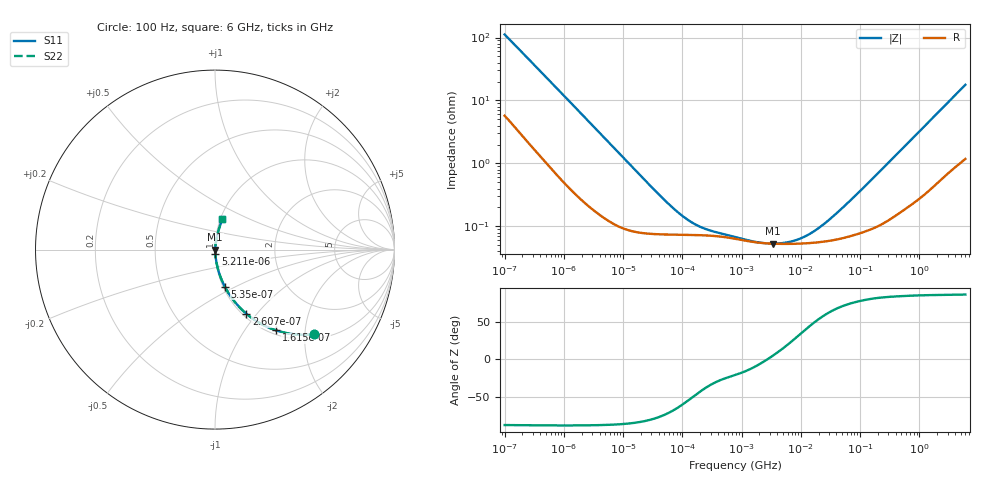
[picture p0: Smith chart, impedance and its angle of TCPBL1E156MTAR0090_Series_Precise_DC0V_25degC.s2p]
! TCPBL1E156MTAR0090 Polymer Tantalum Capacitor Sparameter Model
! Model Generated by Samsung Electro-Mechanics
! Samsung Sparameter Version 5.0
! Date : Oct-10-2024
! Products : Polymer Tantalum Capacitor
! Characteristics :
!  Nominal Capacitance = 15uF
!  Capacitance Tolerance = +/-20%
!  ESR = 90 mohm max at 100kHz
!  Rated Voltage = 25Vdc
!  Size = 1411(unit:inch), 3528(unit:mm)
!  Length = 3.50+/-0.20mm
!  Width = 2.80+/-0.20mm
!  Thickness = 1.10+/-0.10mm
!  Lineup = Conductive Polymer Type
!  Feature = PBL
!  Measurement Temperature : 25degC.
!  DC bias Value = 0V
!  Frequency : 100Hz ~ 6GHz
! External Node Assignments :
!  1  o---||---o  2
# MHz S RI R 50.0
! Freq.  Real(S11)  Im(S11)  Real(S12)  Im(S12)  Real(S21)  Im(S21)  Real(S22)  Im(S22)
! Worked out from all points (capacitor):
!   300 points, 100 Hz to 6 GHz, reference 50 ohm
!   read as one part in series: C = 14.1 uF near 106.2 Hz
!   lowest |Z| = 53.4 mohm at 3.361 MHz (marker M1)
!   series resonance near 2.71 MHz, so ESL is about 240 pH
!   S11 on the Smith chart (normalised r, x): 100 Hz: 1.11, -2.23; 161.5 Hz: 1.07, -1.41; 260.7 Hz: 1.04, -0.89; 535 Hz: 1.02, -0.44; 5.211 kHz: 1.00, -0.05; 6 GHz: 1.02, +0.35
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0.0001  0.5529 -0.4722  0.4471 0.4722  0.4471 0.4722  0.5529 -0.4722
0.0001614771  0.3394 -0.4497  0.6606 0.4497  0.6606 0.4497  0.3394 -0.4497
0.0002607487  0.1752 -0.3577  0.8248 0.3577  0.8248 0.3577  0.1752 -0.3577
0.0003735128  0.0992 -0.2773  0.9008 0.2773  0.9008 0.2773  0.0992 -0.2773
0.0005350431  0.0544 -0.2062  0.9456 0.2062  0.9456 0.2062  0.0544 -0.2062
0.0009739296  0.0197 -0.1197  0.9803 0.1197  0.9803 0.1197  0.0197 -0.1197
0.001998454  0.00625 -0.0602  0.9938 0.0602  0.9938 0.0602  0.00625 -0.0602
0.005210943  0.00185 -0.0236  0.9982 0.0236  0.9982 0.0236  0.00185 -0.0236
0.03993819  0.000759 -0.00314  0.9992 0.00314  0.9992 0.00314  0.000759 -0.00314
0.08700994  0.000739 -0.00146  0.9993 0.00146  0.9993 0.00146  0.000739 -0.00146
0.1583827  0.00073 -0.000824  0.9993 0.000824  0.9993 0.000824  0.00073 -0.000824
0.2883013  0.000714 -0.00049  0.9993 0.00049  0.9993 0.00049  0.000714 -0.00049
0.7981464  0.000633 -0.000234  0.9994 0.000234  0.9994 0.000234  0.000633 -0.000234
1.846192  0.000555 -7.68e-05  0.9994 7.68e-05  0.9994 7.68e-05  0.000555 -7.68e-05
3.360592  0.000532 4.55e-05  0.9995 -4.55e-05  0.9995 -4.55e-05  0.000532 4.55e-05
7.773385  0.000529 0.000269  0.9995 -0.000269  0.9995 -0.000269  0.000529 0.000269
15.95059  0.000549 0.000602  0.9995 -0.000602  0.9995 -0.000602  0.000549 0.000602
25.75656  0.000577 0.000971  0.9994 -0.000971  0.9994 -0.000971  0.000577 0.000971
46.88422  0.000641 0.00173  0.9994 -0.00173  0.9994 -0.00173  0.000641 0.00173
318.7652  0.0014 0.0107  0.9986 -0.0107  0.9986 -0.0107  0.0014 0.0107
1810.813  0.00757 0.0559  0.9924 -0.0559  0.9924 -0.0559  0.00757 0.0559
6000  0.0411 0.1681  0.9589 -0.1681  0.9589 -0.1681  0.0411 0.1681
